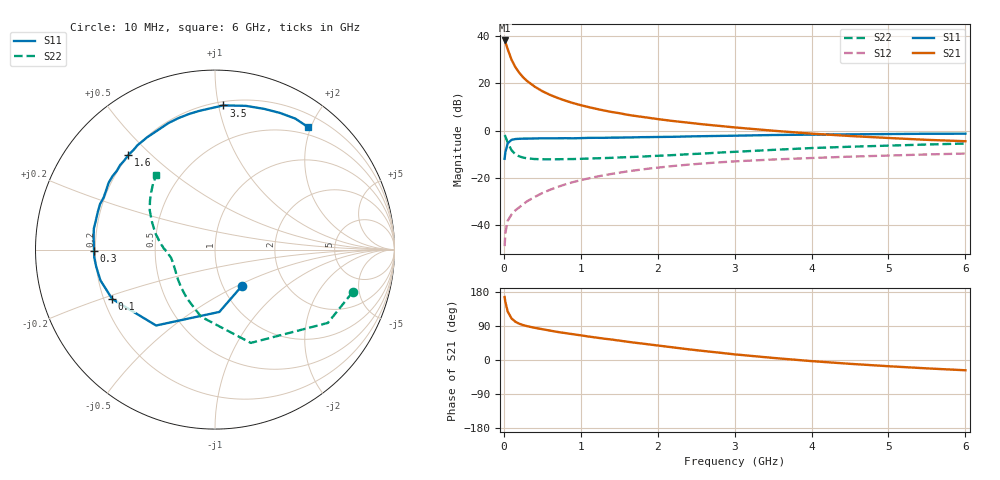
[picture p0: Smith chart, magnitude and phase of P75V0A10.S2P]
! SIEMENS Small Signal Semiconductors
! BFP196
! Si NPN RF Bipolar Junction Transistor in SOT143
! VCE = 5 V  IC = 100 mA
! Common Emitter S-Parameters:  May  1996
# GHz  S  MA  R  50
!  f  S11  S21  S12  S22
! GHz  MAG  ANG  MAG  ANG  MAG  ANG  MAG  ANG
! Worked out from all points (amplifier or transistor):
!   36 points, 10 MHz to 6 GHz, reference 50 ohm
!   highest |S21| = 38.3 dB at 10 MHz (marker M1)
!   |S21| within 3 dB of that: start of sweep to 42.97 MHz
!   unconditionally stable (mu >= 1): 346.6 MHz to 4.838 GHz
!   at 250 MHz: K = 0.93, MSG = 27.0 dB, |S12| = -31.3 dB
!   at 1.4 GHz: K = 1.09, MAG = 11.4 dB, |S12| = -18.4 dB
!   at 6 GHz: K = 0.98, MSG = 2.6 dB, |S12| = -9.8 dB
!   S11 on the Smith chart (normalised r, x): 10 MHz: 1.23, -0.53; 100 MHz: 0.23, -0.22; 300 MHz: 0.19, -0.01; 1.6 GHz: 0.20, +0.43; 3.5 GHz: 0.23, +1.03; 6 GHz: 0.38, +1.95
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0.01  0.2515 -53.0  82.11 166.2  0.0035 77.5  0.8022 -17.2
0.02  0.3481 -86.0  75.59 153.0  0.0067 68.4  0.7498 -33.0
0.05  0.5352 -127.8  53.64 128.1  0.0121 53.6  0.5569 -69.0
0.1  0.6353 -154.3  32.03 109.6  0.0165 50.8  0.3818 -101.8
0.15  0.661 -165.0  22.24 101.0  0.0202 52.7  0.3134 -119.9
0.2  0.6684 -171.6  16.96 95.7  0.0234 57.1  0.2836 -131.6
0.25  0.6741 -176.2  13.57 92.1  0.0271 59.9  0.2664 -140.2
0.3  0.674 -179.4  11.37 89.4  0.0313 62.2  0.258 -145.6
0.4  0.6794 174.5  8.6 85.0  0.0388 64.7  0.2486 -153.6
0.5  0.6851 170.2  6.867 81.3  0.047 65.2  0.246 -158.9
0.6  0.6834 165.9  5.737 77.6  0.0552 65.7  0.2451 -162.4
0.7  0.6859 162.1  4.934 74.0  0.0635 65.4  0.246 -165.0
0.8  0.6888 158.4  4.318 71.0  0.072 64.7  0.2474 -167.0
1.1  0.6998 148.0  3.157 62.0  0.0963 61.8  0.2543 -171.8
1.3  0.7013 141.3  2.678 56.4  0.1124 59.2  0.2603 -174.5
1.6  0.7148 132.4  2.175 48.4  0.1351 54.9  0.2725 -178.0
2.2  0.7373 115.7  1.595 33.3  0.1766 45.6  0.3013 174.4
2.8  0.7698 100.6  1.258 19.4  0.2114 36.5  0.3407 165.4
3.5  0.8047 86.7  0.993 5.5  0.2428 26.4  0.3889 155.3
4.5  0.8308 70.6  0.767 -10.1  0.2793 14.3  0.4536 143.0
5.5  0.8561 58.5  0.635 -22.1  0.3108 3.5  0.5057 132.9
6  0.857 53.0  0.594 -27.1  0.3252 -2.2  0.5302 128.0
